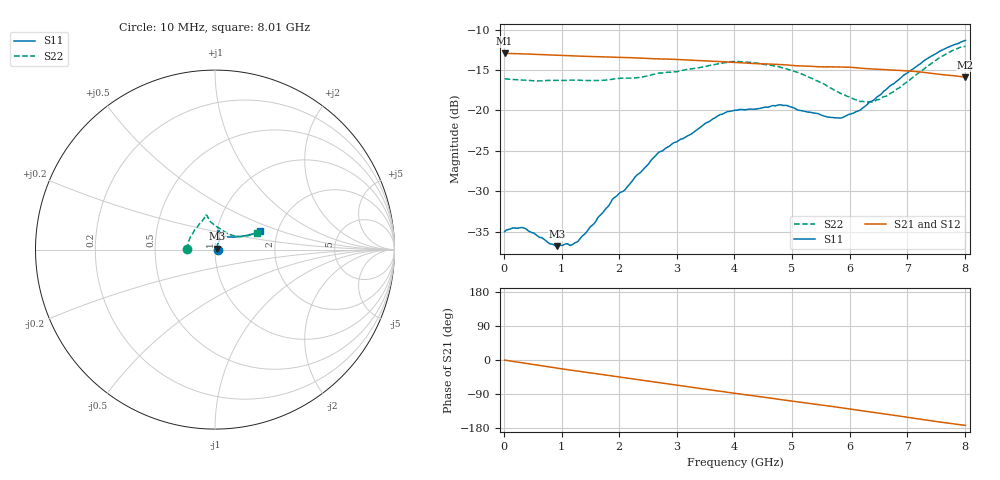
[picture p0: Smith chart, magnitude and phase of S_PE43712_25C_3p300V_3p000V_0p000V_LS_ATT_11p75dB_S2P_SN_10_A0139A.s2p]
! DEVICE ID: PE43712
! File Path: z:\PE43713\PE43713_CHAR_NOM_04292014\AMB\3p300\LS_ATT_11p75dB\PE43713_AMB_3p300V_3p000V_0p000V_LS_ATT_11p75dB_S2P_SN_10_A0139A.s2p
! Serial: 10
! Lot: A0139A
! Temp: 25C
! VDD: 3.300
! VSS: 0.000
! Control_Hi: 3.000
! Control_Lo: 0.000
! Attenuation Step: 11.75dB
! Port 1: RF1
! Port 2: RF2
! ThroughPath:1-2
! IDD: 0.0001471224
! ISS: -7.47e-008
#  Hz  S  RI  R  50
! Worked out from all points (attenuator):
!   801 points, 10 MHz to 8.01 GHz, reference 50 ohm
!   highest |S21| = -12.94 dB at 10 MHz (marker M1); lowest = -15.9 dB at 8.01 GHz (marker M2)
!   lowest |S11| = -36.8 dB at 920 MHz (marker M3), VSWR 1.03, Z = 51.4 + j0.511 ohm
!   |S11| at or under -10 dB: start of sweep to end of sweep
!   |S22| runs from -19.0 to -12.1 dB; largest |S21 - S12| = 0.00081
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1e7  0.0178 0.000294  0.2253 -0.00121  0.2255 -0.00113  -0.1571 0.00108
1.6e8  0.0188 0.000599  0.2241 -0.0155  0.2243 -0.0155  -0.1549 0.0107
3.4e8  0.0188 0.000245  0.221 -0.0321  0.221 -0.0316  -0.1527 0.0199
9.2e8  0.0136 0.00498  0.2041 -0.0803  0.2043 -0.0803  -0.1445 0.0514
1.18e9  0.0116 0.00913  0.1935 -0.099  0.1935 -0.0991  -0.1392 0.0658
1.35e9  0.0117 0.0118  0.186 -0.1107  0.186 -0.1108  -0.1346 0.0739
1.9e9  0.0137 0.0252  0.1571 -0.1445  0.1571 -0.1445  -0.1163 0.1047
2.1e9  0.0145 0.0289  0.1451 -0.1552  0.1451 -0.1551  -0.1104 0.1135
2.68e9  0.0229 0.05  0.1061 -0.1793  0.106 -0.1793  -0.0825 0.1489
3.72e9  0.0235 0.0899  0.0289 -0.1983  0.0287 -0.1983  -0.0555 0.1861
4.01e9  0.0219 0.0978  0.00736 -0.198  0.00734 -0.198  -0.0544 0.193
4.79e9  0.0195 0.1067  -0.0467 -0.1864  -0.0468 -0.1865  -0.041 0.1808
5.35e9  0.03 0.092  -0.0807 -0.1691  -0.0807 -0.169  -0.0255 0.1555
5.64e9  0.0405 0.0813  -0.0966 -0.159  -0.0965 -0.159  -0.00601 0.1395
5.87e9  0.0506 0.0746  -0.11 -0.1493  -0.1099 -0.1493  0.0128 0.126
6.16e9  0.0696 0.0712  -0.1246 -0.1336  -0.1244 -0.1338  0.0412 0.1069
6.3e9  0.0829 0.07  -0.13 -0.1264  -0.1298 -0.1264  0.0569 0.0971
6.42e9  0.0927 0.0698  -0.1346 -0.12  -0.1344 -0.12  0.0696 0.0897
6.68e9  0.1203 0.0709  -0.144 -0.1047  -0.1438 -0.1048  0.0989 0.0776
7.36e9  0.193 0.0838  -0.1595 -0.0604  -0.1594 -0.0604  0.1725 0.0758
7.72e9  0.2283 0.0937  -0.1607 -0.0377  -0.1606 -0.0379  0.2123 0.0849
8.01e9  0.2495 0.1052  -0.1592 -0.0213  -0.159 -0.0215  0.2319 0.09
